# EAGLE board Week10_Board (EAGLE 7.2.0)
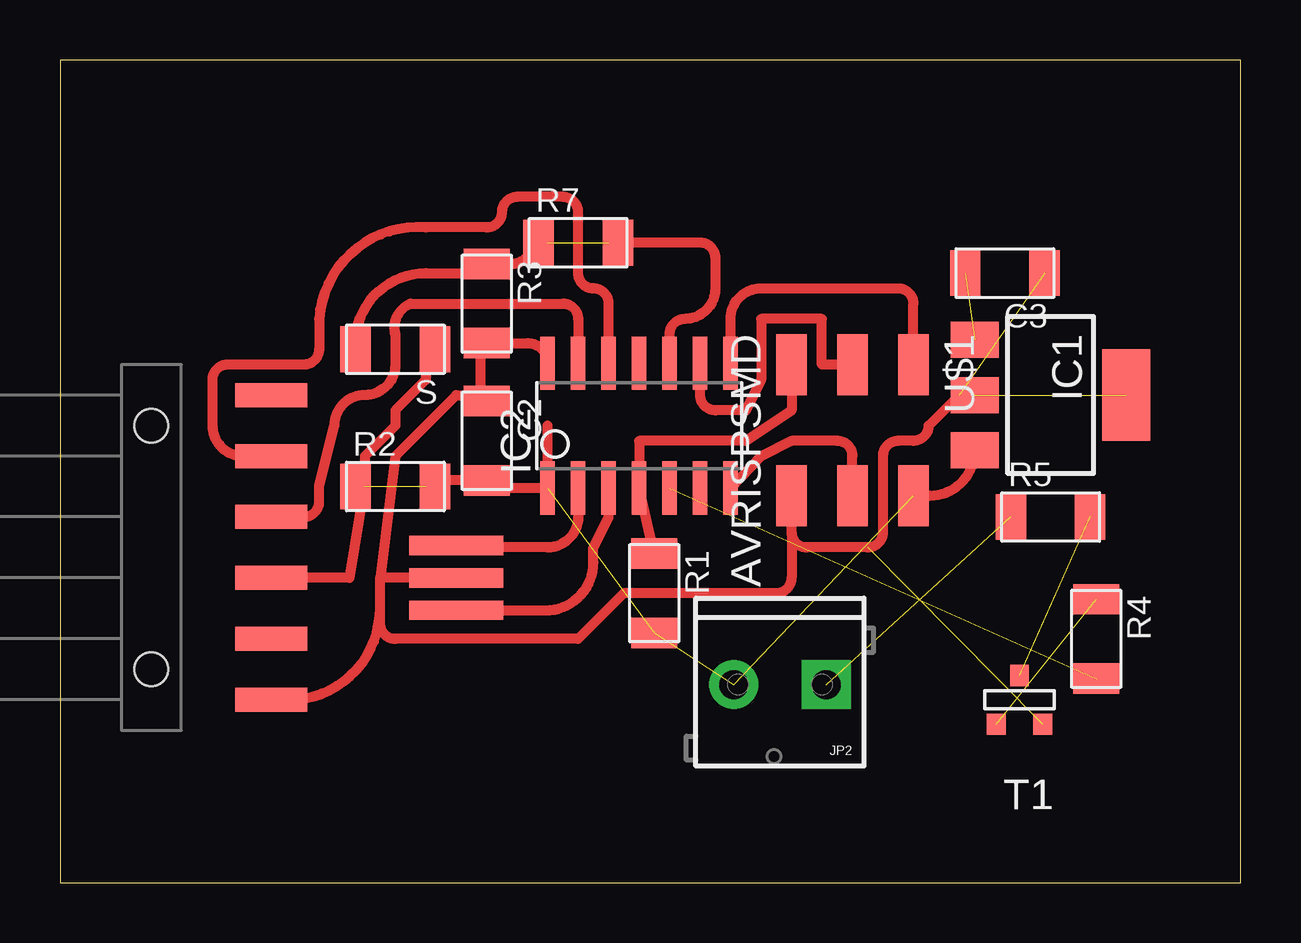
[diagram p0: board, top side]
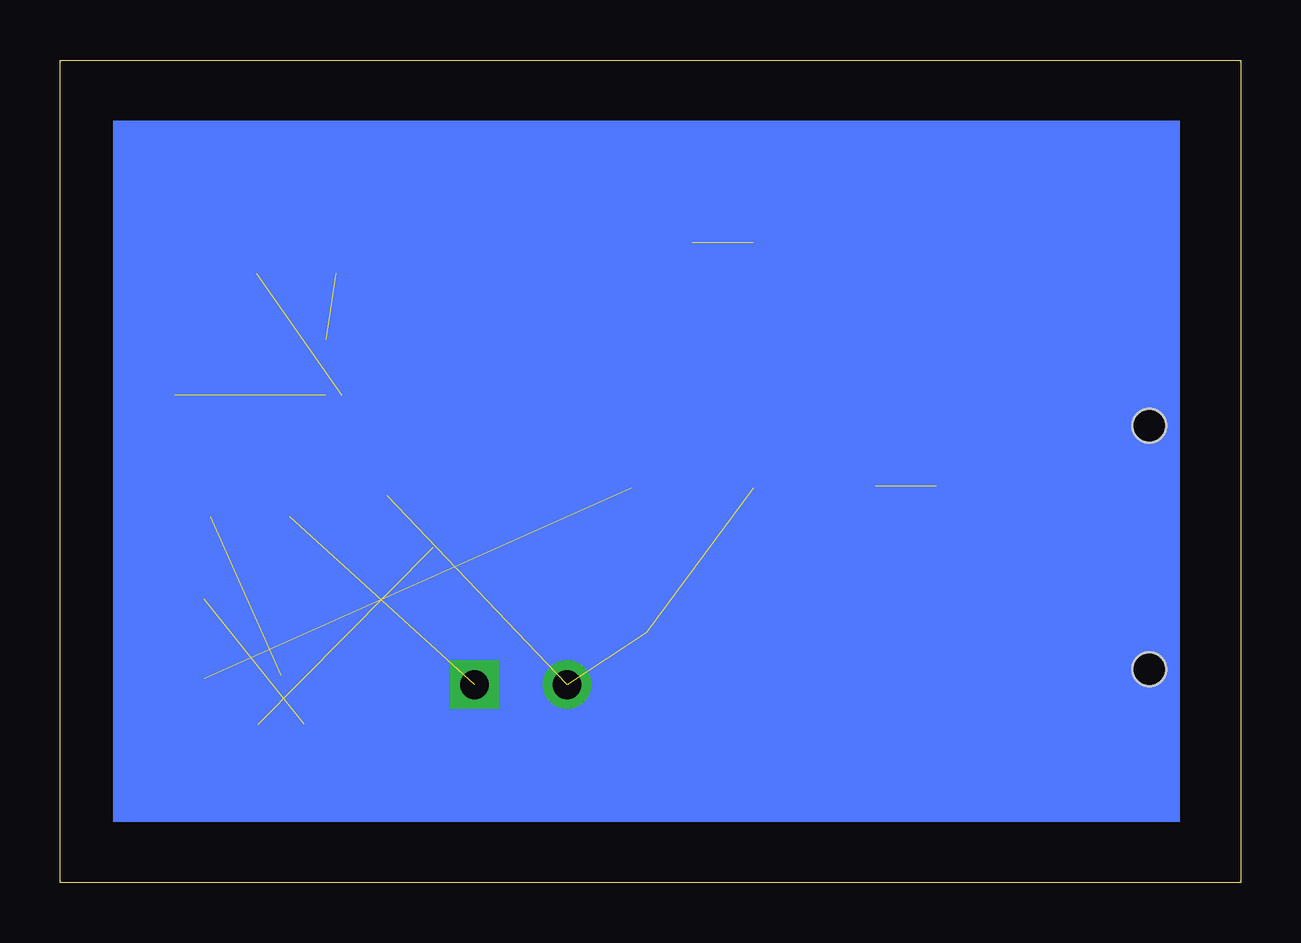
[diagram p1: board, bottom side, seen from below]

Size 49.2 x 34.28 mm. Coordinates in mm from the lower left corner, seen from the top.
Outline: 0,0 49.2,0 49.2,34.28 0,34.28 0,0
Copper layers (1*16): Top 0.035mm / dielectric 1.5mm / Bottom 0.035mm
Design rules "fabmodule": minimum track width 10mil, minimum drill 0.4mm, track to track 0.42mm, track to pad 0.42mm, pad to pad 0.42mm, via to via 0.42mm, smd to smd 0.42mm, copper to edge 40mil, drill to drill 0.8mm, minimum pad ring 10mil, minimum via ring 8mil, stop-mask expansion 4mil, vias tented up to drill 0mil, thermal gap 10mil

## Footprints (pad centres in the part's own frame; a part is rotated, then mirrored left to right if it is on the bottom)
C1206FAB = smd 1.27 x 1.905: 1 -1.651,0; 2 1.651,0
SOT223 = smd 1.5 x 2: 1 -2.3,-3.15; 2 0,-3.15; 3 2.3,-3.15 | smd 3.8 x 2: 4 0,3.15
SOIC14 = smd 0.61 x 2.21: 1 -3.81,-2.603; 2 -2.54,-2.603; 3 -1.27,-2.603; 4 0,-2.603; 5 1.27,-2.603; 6 2.54,-2.603; 7 3.81,-2.603; 8 3.81,2.603; 9 2.54,2.603; 10 1.27,2.603; 11 0,2.603; 12 -1.27,2.603; 13 -2.54,2.603; 14 -3.81,2.603
1X06-SMD = smd 1 x 3: 1 -6.35,5; 2 -3.81,5; 3 -1.27,5; 4 1.27,5; 5 3.81,5; 6 6.35,5 | hole 1.4: -5.08,0; 5.08,0
SCREWTERMINAL-3.5MM-2_LOCK = drill 1.2 pad 2.032 square: 1 -0.178,0 | drill 1.2 pad 2.032: 2 3.678,0
R1206FAB = smd 1.27 x 1.905: 1 -1.651,0; 2 1.651,0
SOT-23 = smd 0.787 x 0.889: 1 0.025,-1.016; 2 -0.94,1.016; 3 0.991,1.016
2X03SMD = smd 2.54 x 1.27: 1 -2.54,2.54; 2 2.92,2.54; 3 -2.54,0; 4 2.92,0; 5 -2.54,-2.54; 6 2.92,-2.54
EFOBM = smd 0.8 x 3.9: 1 -1.35,0; 2 0,0; 3 1.35,0

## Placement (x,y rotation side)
C2  CAP-US1206FAB  [C1206FAB]  17.78,18.41 270 top
C3  CAP-US1206FAB  [C1206FAB]  39.37,25.4 180 top
IC1  5 V  [SOT223]  41.27,20.32 270 top
IC2  ATTINY44-SSU  [SOIC14]  24.13,19.05 0 top
JP1  [1X06-SMD]  3.81,13.97 270 top
JP2  3,8 V  [SCREWTERMINAL-3.5MM-2_LOCK]  31.75,8.25 180 top
R1  10k  [R1206FAB]  24.76,12.06 270 top
R2  0  [R1206FAB]  13.97,16.51 0 top
R3  10k  [R1206FAB]  17.78,24.13 270 top
R4  10k  [R1206FAB]  43.18,10.16 270 top
R5  49.9  [R1206FAB]  41.27,15.24 0 top
R7  0  [R1206FAB]  21.59,26.67 0 top
S  3k  [R1206FAB]  13.97,22.23 180 top
T1  [SOT-23]  40.01,7.62 180 top
U$1  AVRISPSMD  [2X03SMD]  33.02,19.05 270 top
U$3  RESONATOR  [EFOBM]  16.51,12.7 270 top

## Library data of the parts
C2 C3 IC1 IC2 R1-R5 R7 S T1 U$3 = 01_fab
JP1 = SparkFun-Connectors
JP2 = SparkFun-Connectors; PROD_ID: CONN-08399
U$1 = fab

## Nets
GND: C2.1 C3.1 IC1.2 IC1.4 IC2.14 JP1.6 R3.2 T1.2 U$1.6 U$3.2
MISO: IC2.8 U$1.1
MOSI: IC2.7 U$1.4
MOTOR: IC2.5 R4.2
N$1: JP2.1 R5.1
N$2: R5.2 T1.1
N$3: IC2.2 U$3.1
N$4: IC2.3 U$3.3
N$7: C3.2 IC1.1
N$8: R4.1 T1.3
RST: IC2.4 R1.1 U$1.5
RX: IC2.12 JP1.2
SCK: IC2.9 U$1.3
SENSOR: IC2.10 R3.1 S.2
TX: IC2.13 JP1.3
VCC: C2.2 IC1.3 IC2.1 JP1.4 JP2.2 R1.2 S.1 U$1.2

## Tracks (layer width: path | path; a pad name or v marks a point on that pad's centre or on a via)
GND  (3 unrouted)
  Top 0.406: IC1.2 37.46,20.32 36.2,19.05 arc-90 35.56,18.41 34.92,18.41 arc90 34.29,17.78 34.29,14.61 arc-90 33.65,13.97 31.12,13.97 arc-90 30.48,14.61 | 30.48,14.61 U$1.6 | 30.48,14.61 30.48,12.7 arc-90 29.84,12.06 23.49,12.06 21.59,10.16 13.97,10.16 arc-90 13.33,10.8 13.33,11.43 | 13.33,11.43 13.33,12.7 | U$3.2 13.33,12.7 | 17.53,20.32 16.51,20.32 13.97,17.78 13.33,12.7 | 17.53,20.32 C2.1 | 17.53,22.23 R3.2 | 17.53,20.32 17.53,22.23 | 17.53,22.23 arc-90 R3.2 | R3.2 19.49,22.48 arc-90 IC2.14 | JP1.6 9.52,7.62 arc90 13.33,11.43
MISO
  Top 0.406: U$1.1 35.56,24.13 arc90 34.92,24.77 29.21,24.77 arc90 27.94,23.49 IC2.8
MOSI
  Top 0.406: IC2.7 27.88,16.45 | U$1.4 33.02,17.78 arc90 32.38,18.41 30.48,18.41 29.21,17.78 IC2.7 | 27.94,15.88 IC2.7
MOTOR  (1 unrouted)
N$1  (1 unrouted)
N$2  (1 unrouted)
N$3
  Top 0.406: IC2.2 21.59,15.24 arc-90 20.32,13.97 16.59,13.97 arc-90 U$3.1
N$4
  Top 0.406: U$3.3 20.24,11.35 arc90 22.22,13.34 22.22,13.97 22.86,15.24 IC2.3
N$7  (1 unrouted)
N$8  (1 unrouted)
RST
  Top 0.406: R1.1 IC2.4 24.13,18.41 28.57,18.41 30.48,19.69 U$1.5
RX
  Top 0.406: IC2.12 22.86,24.13 arc90 22.22,24.77 arc-90 21.59,25.4 21.59,27.94 arc90 20.95,28.58 19.05,28.58 arc90 18.41,27.94 arc-90 17.78,27.3 15.24,27.3 arc90 10.79,23.49 10.79,22.23 arc-90 10.16,21.59 6.98,21.59 arc90 6.35,20.95 6.35,19.05 arc90 7.62,17.78 JP1.2 | 9.52,17.78 JP1.2 | 8.89,17.78 JP1.2
SCK
  Top 0.406: U$1.3 31.75,21.59 31.75,23.49 29.21,23.49 29.21,20.95 28.57,19.69 27.3,19.69 arc-90 26.67,20.32 IC2.9
SENSOR  (1 unrouted)
  Top 0.406: S.2 12.32,22.48 arc-90 15.24,25.4 17.4,25.4 arc90 R3.1 18.8,25.78 arc90 19.68,26.67 20.32,26.67 | IC2.10 25.4,22.86 arc-90 26.03,23.49 arc90 27.3,24.77 27.3,26.04 arc90 26.67,26.67 22.86,26.67
TX
  Top 0.406: JP1.3 10.16,15.24 arc90 10.79,15.88 10.79,16.51 11.43,19.05 arc-90 12.7,20.32 arc90 13.97,21.59 13.97,22.86 arc-82 14.6,24.13 20.95,24.13 arc-90 21.59,23.49 IC2.13
VCC  (4 unrouted)
  Top 0.406: JP1.4 12.06,12.7 12.7,16.51 12.7,17.78 13.97,19.05 13.97,19.69 15.24,20.95 15.24,22.23 15.62,21.97 S.1 | U$1.2 36.23,16.13 arc90 IC1.3 | 24.38,10.16 arc-90 R1.2 | 20.32,19.05 IC2.1 18.1,16.45 C2.2 15.49,16.76 arc90 15.24,16.51
(copper drawn outside any net)
  shapes: Bottom area x1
